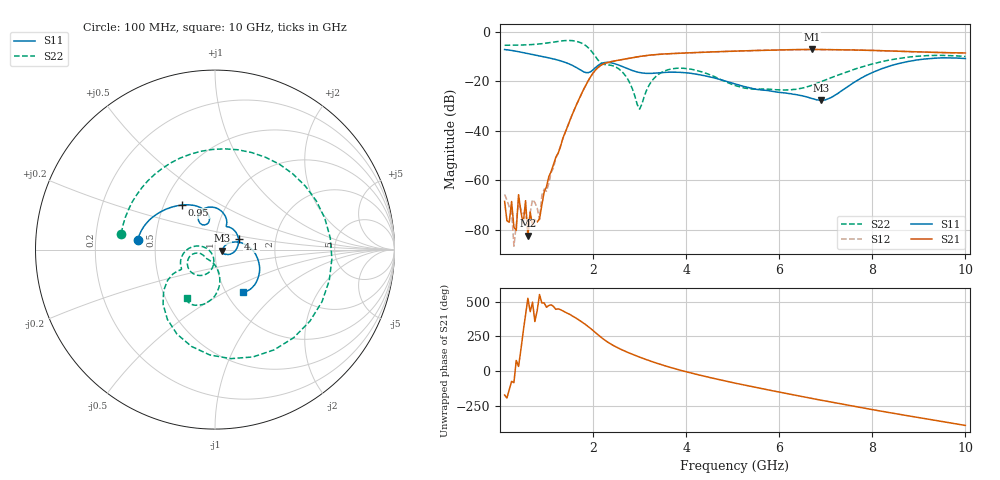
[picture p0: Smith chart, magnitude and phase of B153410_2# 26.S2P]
!  2-Port S-parameters saved by WinCal
! VAR MeasName=S-Parameters (CALIBRATED_DATA) read from VNA (N5245A)
! VAR MeasDate=2016-12-23 10:00:41
! VAR NAME=B153410_2# 26
! VAR FILENAME=B153410_2# 26.S2P
! VAR DATE=2016-12-23 10:00:41
! VAR PHYS_PORTS=1,2
# Hz S DB R 50
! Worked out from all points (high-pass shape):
!   199 points, 100 MHz to 10 GHz, reference 50 ohm
!   highest |S21| = -7.21 dB at 6.7 GHz (marker M1); lowest = -82.5 dB at 600 MHz (marker M2)
!   |S21| within 3 dB of the highest: 2.944 GHz to end of sweep
!   lowest |S11| = -27.7 dB at 6.9 GHz (marker M3), VSWR 1.09, Z = 54.3 - j0.552 ohm
!   |S11| at or under -10 dB: 902.4 MHz to end of sweep
!   |S22| runs from -31.3 to -3.6 dB; largest |S21 - S12| = 0.0044
!   S11 on the Smith chart (normalised r, x): 100 MHz: 0.40, +0.05; 950 MHz: 0.62, +0.34; 4.1 GHz: 1.29, +0.16; 10 GHz: 1.20, -0.62
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1e8  -7.24 172.6  -68.55 -168.9  -65.74 -27.0  -5.51 170.3
2e8  -7.46 165.6  -76.97 -129.7  -70.79 -87.9  -5.50 160.3
2.5e8  -7.59 162.2  -68.59 -71.4  -72.33 -178.1  -5.50 155.4
3.5e8  -7.92 156.0  -80.24 78.2  -78.08 -32.3  -5.48 145.0
4e8  -8.10 153.1  -65.86 35.6  -67.94 -29.7  -5.45 139.8
5e8  -8.48 147.7  -77.63 -73.7  -73.53 116.4  -5.39 128.8
5.5e8  -8.67 145.2  -68.27 47.3  -72.90 -15.4  -5.36 123.1
6e8  -8.86 142.7  -82.46 163.0  -80.59 -106.6  -5.32 117.2
7e8  -9.23 138.0  -78.36 136.1  -67.82 -89.4  -5.21 104.8
8.5e8  -9.80 131.1  -75.62 -169.6  -75.85 -177.9  -4.98 84.4
9.5e8  -10.18 126.7  -64.79 130.2  -63.58 137.7  -4.76 69.4
1.35e9  -12.09 109.3  -43.14 73.4  -43.29 73.7  -3.70 -4.5
1.75e9  -15.73 101.2  -25.21 -3.6  -25.22 -3.4  -4.62 -92.8
2.65e9  -14.26 72.6  -11.19 150.1  -11.21 150.1  -16.72 177.3
3e9  -16.52 65.0  -10.03 102.3  -10.05 102.2  -31.29 -141.7
3.4e9  -16.65 59.3  -9.19 55.2  -9.21 55.4  -17.34 -106.5
4.1e9  -16.82 24.7  -8.53 -10.9  -8.55 -10.8  -15.16 -151.9
5.05e9  -21.12 -17.2  -7.86 -83.9  -7.88 -83.6  -21.75 -163.6
6.7e9  -27.00 -19.0  -7.21 166.4  -7.23 166.5  -21.67 -92.2
6.9e9  -27.72 -7.1  -7.22 153.7  -7.24 153.8  -20.18 -85.9
8.35e9  -14.05 2.3  -7.81 66.0  -7.82 66.3  -11.54 -91.3
1e10  -10.87 -56.4  -8.62 -27.2  -8.62 -26.6  -10.06 -120.2
